| licensed IBIS model.
| 10.This license is subject to the laws of the state of Texas, USA, without
| regard for its conflicts of laws provisions.
[IBIS ver] 3.2
[File name] efr32xg23_qfn40_hfclkout.ibs
[File Rev] 1.0
[Date]  Oct 26, 2021
[Source] File originated at Silicon Labs Inc.
[Notes]  1. MIN TYP MAX information is based on Temperature and Voltage
   characteristics only.
   2. The model of I/O buffer has the mode of input, input w/ pull-
   down resistor, input w/ pull-up resistor, pushpull, wiredor,
   wiredor w/ pull-down resistor, wiredand, wiredand w/ pull-up
   resistor.
   3. Supply voltages modelled are 1.8V, 3.0V and 3.3V.
   4. Slew rate of buffer can be typ (sr4), min (sr0), max (sr7).
[Disclaimer]
| READ THE TERMS OF THIS LICENSE BEFORE USING THIS IBIS MODEL. IF YOU DO
| NOT ACCEPT THE TERMS OF THIS LICENSE, YOU ARE NOT PERMITTED TO USE THIS
| IBIS MODEL.
| Silicon Laboratories Inc. ("Silicon Labs") is the exclusive owner of this
| IBIS model,  and hereby grants to Licensee a limited, non-exclusive,
| worldwide, royalty-free, non-transferable, perpetual license to use this
| IBIS model, subject to the following terms and conditions:
| 1.If you are using this IBIS model for the benefit of your employer,
| then your acceptance of these terms will be considered an acceptance by
| your employer and your employer will be deemed to be the Licensee of this
| IBIS model.
| 2.Licensee is granted this license to use this IBIS model only for the
| purpose  modeling input/output buffers of Silicon Labs integrated circuits,
| and is not granted any rights to sell, load, rent, lease or license this
| IBIS model in whole or in part, or in modified form, to any third party.
| 3.Licensee may modify this IBIS model to suit its specific applications,
| but rights to derivative works and such modifications, including all
| intellectual property rights, shall belong exclusively to Silicon Labs. To
| the extent that Silicon Labs is not the owner of such modifications or
| derivatives, Licensee hereby grants to Silicon Labs a non-exclusive,
| worldwide, royalty-free, fully-transferable, assignable, perpetual license
| to use, copy, modify, make derivatives, sell, offer to sell, make, have
| made and sub-license such derivative and modifications in any manner, for
| any purpose, with no accounting to Licensee.
| 4.This IBIS model is provided on an "AS IS" basis and Silicon Labs makes
| no representations or warranties with respect to the information contained
| in this IBIS model.
| 5.SILICON LABS DISCLAIMS AND LICENSEE WAIVES ALL WARRANTIES, EXPRESS OR
| IMPLIED, INCLUDING WARRANTIES OF MERCHANTABILITY, NON-INFRINGEMENT AND
| FITNESS FOR A PARTICULAR PURPOSE.
| 6.The entire risk as to quality and performance is with Licensee.
| ACCORDINGLY, IN NO EVENT SHALL SILICON LABS BE LIABLE FOR ANY DAMAGES,
| WHETHER IN CONTRACT OR TORT, INCLUDING ANY LOST PROFITS OR OTHER INCIDENTAL,
| CONSEQUENTIAL, EXEMPLARY, OR PUNITIVE DAMAGES ARISING OUT OF THE USE OR
| APPLICATION OF THIS IBIS MODEL.
| 7.Silicon Labs reserves the right to make changes without notice to this
| IBIS model to improve reliability, function, or design.
| 8.Silicon Labs does not convey any license under patent rights or any other
| intellectual property rights, including those of third parties.
| 9.Silicon Labs is not obligated to provide maintenance or support for the
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[Copyright] Copyright 2021 Silicon Labs Inc.
|   Component 40nm General Purpose
[Component] Ocelot
[Manufacturer] Silicon Labs Inc.
[Package]
| QFN40
| variable   typ   min   max
R_pkg   0.467   0.424   0.495
L_pkg   1.57E-09	8.37E-10	2.02E-09
C_pkg   2.59E-13	1.87E-13	4.17E-13
[Pin]	signal_name	model_name	R_pin   L_pin   C_pin
1	PC00   gpio_lcd	0.477   1.72E-09	2.59E-13
2	PC01   gpio_lcd	0.466   1.55E-09	2.45E-13
3	PC02   gpio_lcd	0.456   1.38E-09	2.31E-13
4	PC03   gpio_lcd	0.454   1.34E-09	2.28E-13
5	PC04   gpio_lcd	0.452   1.31E-09	2.25E-13
6	PC05   gpio_lcd	0.458   1.42E-09	2.34E-13
7	PC06   gpio_lcd	0.470   1.61E-09	2.50E-13
8	HFCLKOUT	NC   0.453   1.32E-09	2.27E-13
9	HFXTAL_I	NC   0.455   1.36E-09	2.30E-13
10	HFXTAL_O	NC   0.463   1.49E-09	2.40E-13
11	RESETn   NC   0.463   1.49E-09	2.40E-13
12	RFVDD   NC   0.459   1.43E-09	2.35E-13
13	RFVSS   NC   0.424   8.37E-10	1.87E-13
14	SUBG_I1   NC   0.455   1.35E-09	2.29E-13
15	SUBG_I0   NC   0.456   1.37E-09	2.31E-13
16	SUBG_O1   NC   0.459   1.43E-09	2.35E-13
17	SUBG_O0   NC   0.464   1.51E-09	2.42E-13
18	PAVDD   NC   0.470   1.62E-09	2.50E-13
19	PB01   gpio_lcd	0.467   1.55E-09	2.45E-13
20	PB00   gpio_lcd	0.480   1.78E-09	2.63E-13
21	PA00   gpio_lcd	0.487   1.89E-09	2.72E-13
22	PA01   gpio_lcd	0.476   1.71E-09	2.58E-13
23	PA02   gpio_3v   0.472   1.64E-09	2.53E-13
24	PA03   gpio_3v   0.473   1.66E-09	2.54E-13
25	PA04   gpio_lcd	0.479   1.77E-09	2.62E-13
26	PA05   gpio_lcd	0.491   1.95E-09	2.78E-13
27	PA06   gpio_lcd	0.473   1.66E-09	2.54E-13
28	PA07   gpio_lcd	0.479   1.76E-09	2.62E-13
29	PA08   gpio_lcd	0.489   1.93E-09	2.76E-13
30	DECOUPLE	NC   0.495   2.02E-09	2.83E-13
31	VREGSW   NC   0.451   1.29E-09	4.17E-13
32	VREGVDD 	NC   0.446   1.21E-09	3.91E-13
33	VREGVSS   NC   0.442   1.15E-09	3.70E-13
34	DVDD   NC   0.477   1.73E-09	2.60E-13
35	AVDD   NC   0.475   1.70E-09	2.57E-13
36	IOVDD   NC   0.478   1.75E-09	2.61E-13
37	PD03   gpio_lcd	0.476   1.71E-09	2.58E-13
38	PD02   gpio_lcd	0.476   1.70E-09	2.58E-13
39	PD01   gpio_3v   0.477   1.73E-09	2.60E-13
40	PD00   gpio_3v   0.482   1.82E-09	2.67E-13
| End of package information
[Component]   gpio_lcd
[Manufacturer]   Silicon Labs Inc.
[Package]
|  variable   typ   min   max
R_pkg   0   0   0
L_pkg   0   0   0
C_pkg   0   0   0
[Pin]   signal_name   model_name   R_pin   L_pin   C_pin
vdd   vddio   POWER
pad   pad   gpio_lcd
gnd   gndio   GND
[Model Selector] gpio_lcd
lcd_input_1p8V_sr0  1.8V, input mode, MODEn=0/1, slew_rate=0, SLEWRATE[ALT]=0
lcd_input_1p8V_sr4  1.8V, input mode, MODEn=0/1, slew_rate=4, SLEWRATE[ALT]=4
lcd_input_1p8V_sr7  1.8V, input mode, MODEn=0/1, slew_rate=7, SLEWRATE[ALT]=7
lcd_input_3p0V_sr0  3.0V, input mode, MODEn=0/1, slew_rate=0, SLEWRATE[ALT]=0
lcd_input_3p0V_sr4  3.0V, input mode, MODEn=0/1, slew_rate=4, SLEWRATE[ALT]=4
lcd_input_3p0V_sr7  3.0V, input mode, MODEn=0/1, slew_rate=7, SLEWRATE[ALT]=7
lcd_input_3p3V_sr0  3.3V, input mode, MODEn=0/1, slew_rate=0, SLEWRATE[ALT]=0
lcd_input_3p3V_sr4  3.3V, input mode, MODEn=0/1, slew_rate=4, SLEWRATE[ALT]=4
lcd_input_3p3V_sr7  3.3V, input mode, MODEn=0/1, slew_rate=7, SLEWRATE[ALT]=7
lcd_inputpd_1p8V_sr0  1.8V, input mode with pull-down res, MODEn=2/3, slew_rate=0, SLEWRATE[ALT]=0
lcd_inputpd_1p8V_sr4  1.8V, input mode with pull-down res, MODEn=2/3, slew_rate=4, SLEWRATE[ALT]=4
lcd_inputpd_1p8V_sr7  1.8V, input mode with pull-down res, MODEn=2/3, slew_rate=7, SLEWRATE[ALT]=7
lcd_inputpd_3p0V_sr0  3.0V, input mode with pull-down res, MODEn=2/3, slew_rate=0, SLEWRATE[ALT]=0
lcd_inputpd_3p0V_sr4  3.0V, input mode with pull-down res, MODEn=2/3, slew_rate=4, SLEWRATE[ALT]=4
lcd_inputpd_3p0V_sr7  3.0V, input mode with pull-down res, MODEn=2/3, slew_rate=7, SLEWRATE[ALT]=7
lcd_inputpd_3p3V_sr0  3.3V, input mode with pull-down res, MODEn=2/3, slew_rate=0, SLEWRATE[ALT]=0
lcd_inputpd_3p3V_sr4  3.3V, input mode with pull-down res, MODEn=2/3, slew_rate=4, SLEWRATE[ALT]=4
lcd_inputpd_3p3V_sr7  3.3V, input mode with pull-down res, MODEn=2/3, slew_rate=7, SLEWRATE[ALT]=7
lcd_inputpu_1p8V_sr0  1.8V, input mode with pull-up res, MODEn=2/3, slew_rate=0, SLEWRATE[ALT]=0
lcd_inputpu_1p8V_sr4  1.8V, input mode with pull-up res, MODEn=2/3, slew_rate=4, SLEWRATE[ALT]=4
lcd_inputpu_1p8V_sr7  1.8V, input mode with pull-up res, MODEn=2/3, slew_rate=7, SLEWRATE[ALT]=7
lcd_inputpu_3p0V_sr0  3.0V, input mode with pull-up res, MODEn=2/3, slew_rate=0, SLEWRATE[ALT]=0
lcd_inputpu_3p0V_sr4  3.0V, input mode with pull-up res, MODEn=2/3, slew_rate=4, SLEWRATE[ALT]=4
lcd_inputpu_3p0V_sr7  3.0V, input mode with pull-up res, MODEn=2/3, slew_rate=7, SLEWRATE[ALT]=7
lcd_inputpu_3p3V_sr0  3.3V, input mode with pull-up res, MODEn=2/3, slew_rate=0, SLEWRATE[ALT]=0
lcd_inputpu_3p3V_sr4  3.3V, input mode with pull-up res, MODEn=2/3, slew_rate=4, SLEWRATE[ALT]=4
lcd_inputpu_3p3V_sr7  3.3V, input mode with pull-up res, MODEn=2/3, slew_rate=7, SLEWRATE[ALT]=7
lcd_pushpull_1p8V_sr0  1.8V, pushpull mode, MODEn=4/5, slew_rate=0, SLEWRATE[ALT]=0
lcd_pushpull_1p8V_sr4  1.8V, pushpull mode, MODEn=4/5, slew_rate=4, SLEWRATE[ALT]=4
lcd_pushpull_1p8V_sr7  1.8V, pushpull mode, MODEn=4/5, slew_rate=7, SLEWRATE[ALT]=7
lcd_pushpull_3p0V_sr0  3.0V, pushpull mode, MODEn=4/5, slew_rate=0, SLEWRATE[ALT]=0
lcd_pushpull_3p0V_sr4  3.0V, pushpull mode, MODEn=4/5, slew_rate=4, SLEWRATE[ALT]=4
lcd_pushpull_3p0V_sr7  3.0V, pushpull mode, MODEn=4/5, slew_rate=7, SLEWRATE[ALT]=7
lcd_pushpull_3p3V_sr0  3.3V, pushpull mode, MODEn=4/5, slew_rate=0, SLEWRATE[ALT]=0
lcd_pushpull_3p3V_sr4  3.3V, pushpull mode, MODEn=4/5, slew_rate=4, SLEWRATE[ALT]=4
lcd_pushpull_3p3V_sr7  3.3V, pushpull mode, MODEn=4/5, slew_rate=7, SLEWRATE[ALT]=7
lcd_wiredor_1p8V_sr0  1.8V, open-source mode, MODEn=6, slew_rate=0, SLEWRATE[ALT]=0
lcd_wiredor_1p8V_sr4  1.8V, open-source mode, MODEn=6, slew_rate=4, SLEWRATE[ALT]=4
lcd_wiredor_1p8V_sr7  1.8V, open-source mode, MODEn=6, slew_rate=7, SLEWRATE[ALT]=7
lcd_wiredor_3p0V_sr0  3.0V, open-source mode, MODEn=6, slew_rate=0, SLEWRATE[ALT]=0
lcd_wiredor_3p0V_sr4  3.0V, open-source mode, MODEn=6, slew_rate=4, SLEWRATE[ALT]=4
lcd_wiredor_3p0V_sr7  3.0V, open-source mode, MODEn=6, slew_rate=7, SLEWRATE[ALT]=7
lcd_wiredor_3p3V_sr0  3.3V, open-source mode, MODEn=6, slew_rate=0, SLEWRATE[ALT]=0
lcd_wiredor_3p3V_sr4  3.3V, open-source mode, MODEn=6, slew_rate=4, SLEWRATE[ALT]=4
lcd_wiredor_3p3V_sr7  3.3V, open-source mode, MODEn=6, slew_rate=7, SLEWRATE[ALT]=7
lcd_wiredorpd_1p8V_sr0  1.8V, open-source mode with pull-down res, MODEn=7, slew_rate=0, SLEWRATE[ALT]=0
lcd_wiredorpd_1p8V_sr4  1.8V, open-source mode with pull-down res, MODEn=7, slew_rate=4, SLEWRATE[ALT]=4
lcd_wiredorpd_1p8V_sr7  1.8V, open-source mode with pull-down res, MODEn=7, slew_rate=7, SLEWRATE[ALT]=7
lcd_wiredorpd_3p0V_sr0  3.0V, open-source mode with pull-down res, MODEn=7, slew_rate=0, SLEWRATE[ALT]=0
lcd_wiredorpd_3p0V_sr4  3.0V, open-source mode with pull-down res, MODEn=7, slew_rate=4, SLEWRATE[ALT]=4
lcd_wiredorpd_3p0V_sr7  3.0V, open-source mode with pull-down res, MODEn=7, slew_rate=7, SLEWRATE[ALT]=7
lcd_wiredorpd_3p3V_sr0  3.3V, open-source mode with pull-down res, MODEn=7, slew_rate=0, SLEWRATE[ALT]=0
lcd_wiredorpd_3p3V_sr4  3.3V, open-source mode with pull-down res, MODEn=7, slew_rate=4, SLEWRATE[ALT]=4
lcd_wiredorpd_3p3V_sr7  3.3V, open-source mode with pull-down res, MODEn=7, slew_rate=7, SLEWRATE[ALT]=7
lcd_wiredand_1p8V_sr0  1.8V, open-drain mode, MODEn=8/9/12/13, slew_rate=0, SLEWRATE[ALT]=0
lcd_wiredand_1p8V_sr4  1.8V, open-drain mode, MODEn=8/9/12/13, slew_rate=4, SLEWRATE[ALT]=4
lcd_wiredand_1p8V_sr7  1.8V, open-drain mode, MODEn=8/9/12/13, slew_rate=7, SLEWRATE[ALT]=7
lcd_wiredand_3p0V_sr0  3.0V, open-drain mode, MODEn=8/9/12/13, slew_rate=0, SLEWRATE[ALT]=0
lcd_wiredand_3p0V_sr4  3.0V, open-drain mode, MODEn=8/9/12/13, slew_rate=4, SLEWRATE[ALT]=4
lcd_wiredand_3p0V_sr7  3.0V, open-drain mode, MODEn=8/9/12/13, slew_rate=7, SLEWRATE[ALT]=7
lcd_wiredand_3p3V_sr0  3.3V, open-drain mode, MODEn=8/9/12/13, slew_rate=0, SLEWRATE[ALT]=0
lcd_wiredand_3p3V_sr4  3.3V, open-drain mode, MODEn=8/9/12/13, slew_rate=4, SLEWRATE[ALT]=4
lcd_wiredand_3p3V_sr7  3.3V, open-drain mode, MODEn=8/9/12/13, slew_rate=7, SLEWRATE[ALT]=7
lcd_wiredandpu_1p8V_sr0  1.8V, open-drain mode with pull-up res, MODEn=10/11/14/15, slew_rate=0, SLEWRATE[ALT]=0
lcd_wiredandpu_1p8V_sr4  1.8V, open-drain mode with pull-up res, MODEn=10/11/14/15, slew_rate=4, SLEWRATE[ALT]=4
lcd_wiredandpu_1p8V_sr7  1.8V, open-drain mode with pull-up res, MODEn=10/11/14/15, slew_rate=7, SLEWRATE[ALT]=7
lcd_wiredandpu_3p0V_sr0  3.0V, open-drain mode with pull-up res, MODEn=10/11/14/15, slew_rate=0, SLEWRATE[ALT]=0
lcd_wiredandpu_3p0V_sr4  3.0V, open-drain mode with pull-up res, MODEn=10/11/14/15, slew_rate=4, SLEWRATE[ALT]=4
lcd_wiredandpu_3p0V_sr7  3.0V, open-drain mode with pull-up res, MODEn=10/11/14/15, slew_rate=7, SLEWRATE[ALT]=7
lcd_wiredandpu_3p3V_sr0  3.3V, open-drain mode with pull-up res, MODEn=10/11/14/15, slew_rate=0, SLEWRATE[ALT]=0
lcd_wiredandpu_3p3V_sr4  3.3V, open-drain mode with pull-up res, MODEn=10/11/14/15, slew_rate=4, SLEWRATE[ALT]=4
lcd_wiredandpu_3p3V_sr7  3.3V, open-drain mode with pull-up res, MODEn=10/11/14/15, slew_rate=7, SLEWRATE[ALT]=7
[Component]   gpio_3v
[Manufacturer]   Silicon Labs Inc.
[Package]
|  variable   typ   min   max
R_pkg   0   0   0
L_pkg   0   0   0
C_pkg   0   0   0
[Pin]   signal_name   model_name   R_pin   L_pin   C_pin
vdd   vddio   POWER
pad   pad   gpio_3v
gnd   gndio   GND
[Model Selector] gpio_3v
3v_input_1p8V_sr0  1.8V, input mode, MODEn=0/1, slew_rate=0, SLEWRATE[ALT]=0
3v_input_1p8V_sr4  1.8V, input mode, MODEn=0/1, slew_rate=4, SLEWRATE[ALT]=4
3v_input_1p8V_sr7  1.8V, input mode, MODEn=0/1, slew_rate=7, SLEWRATE[ALT]=7
3v_input_3p0V_sr0  3.0V, input mode, MODEn=0/1, slew_rate=0, SLEWRATE[ALT]=0
3v_input_3p0V_sr4  3.0V, input mode, MODEn=0/1, slew_rate=4, SLEWRATE[ALT]=4
3v_input_3p0V_sr7  3.0V, input mode, MODEn=0/1, slew_rate=7, SLEWRATE[ALT]=7
3v_input_3p3V_sr0  3.3V, input mode, MODEn=0/1, slew_rate=0, SLEWRATE[ALT]=0
3v_input_3p3V_sr4  3.3V, input mode, MODEn=0/1, slew_rate=4, SLEWRATE[ALT]=4
3v_input_3p3V_sr7  3.3V, input mode, MODEn=0/1, slew_rate=7, SLEWRATE[ALT]=7
3v_inputpd_1p8V_sr0  1.8V, input mode with pull-down res, MODEn=2/3, slew_rate=0, SLEWRATE[ALT]=0
3v_inputpd_1p8V_sr4  1.8V, input mode with pull-down res, MODEn=2/3, slew_rate=4, SLEWRATE[ALT]=4
3v_inputpd_1p8V_sr7  1.8V, input mode with pull-down res, MODEn=2/3, slew_rate=7, SLEWRATE[ALT]=7
3v_inputpd_3p0V_sr0  3.0V, input mode with pull-down res, MODEn=2/3, slew_rate=0, SLEWRATE[ALT]=0
3v_inputpd_3p0V_sr4  3.0V, input mode with pull-down res, MODEn=2/3, slew_rate=4, SLEWRATE[ALT]=4
3v_inputpd_3p0V_sr7  3.0V, input mode with pull-down res, MODEn=2/3, slew_rate=7, SLEWRATE[ALT]=7
3v_inputpd_3p3V_sr0  3.3V, input mode with pull-down res, MODEn=2/3, slew_rate=0, SLEWRATE[ALT]=0
3v_inputpd_3p3V_sr4  3.3V, input mode with pull-down res, MODEn=2/3, slew_rate=4, SLEWRATE[ALT]=4
3v_inputpd_3p3V_sr7  3.3V, input mode with pull-down res, MODEn=2/3, slew_rate=7, SLEWRATE[ALT]=7
3v_inputpu_1p8V_sr0  1.8V, input mode with pull-up res, MODEn=2/3, slew_rate=0, SLEWRATE[ALT]=0
3v_inputpu_1p8V_sr4  1.8V, input mode with pull-up res, MODEn=2/3, slew_rate=4, SLEWRATE[ALT]=4
3v_inputpu_1p8V_sr7  1.8V, input mode with pull-up res, MODEn=2/3, slew_rate=7, SLEWRATE[ALT]=7
3v_inputpu_3p0V_sr0  3.0V, input mode with pull-up res, MODEn=2/3, slew_rate=0, SLEWRATE[ALT]=0
3v_inputpu_3p0V_sr4  3.0V, input mode with pull-up res, MODEn=2/3, slew_rate=4, SLEWRATE[ALT]=4
3v_inputpu_3p0V_sr7  3.0V, input mode with pull-up res, MODEn=2/3, slew_rate=7, SLEWRATE[ALT]=7
3v_inputpu_3p3V_sr0  3.3V, input mode with pull-up res, MODEn=2/3, slew_rate=0, SLEWRATE[ALT]=0
3v_inputpu_3p3V_sr4  3.3V, input mode with pull-up res, MODEn=2/3, slew_rate=4, SLEWRATE[ALT]=4
3v_inputpu_3p3V_sr7  3.3V, input mode with pull-up res, MODEn=2/3, slew_rate=7, SLEWRATE[ALT]=7
3v_pushpull_1p8V_sr0  1.8V, pushpull mode, MODEn=4/5, slew_rate=0, SLEWRATE[ALT]=0
3v_pushpull_1p8V_sr4  1.8V, pushpull mode, MODEn=4/5, slew_rate=4, SLEWRATE[ALT]=4
3v_pushpull_1p8V_sr7  1.8V, pushpull mode, MODEn=4/5, slew_rate=7, SLEWRATE[ALT]=7
3v_pushpull_3p0V_sr0  3.0V, pushpull mode, MODEn=4/5, slew_rate=0, SLEWRATE[ALT]=0
3v_pushpull_3p0V_sr4  3.0V, pushpull mode, MODEn=4/5, slew_rate=4, SLEWRATE[ALT]=4
3v_pushpull_3p0V_sr7  3.0V, pushpull mode, MODEn=4/5, slew_rate=7, SLEWRATE[ALT]=7
3v_pushpull_3p3V_sr0  3.3V, pushpull mode, MODEn=4/5, slew_rate=0, SLEWRATE[ALT]=0
3v_pushpull_3p3V_sr4  3.3V, pushpull mode, MODEn=4/5, slew_rate=4, SLEWRATE[ALT]=4
3v_pushpull_3p3V_sr7  3.3V, pushpull mode, MODEn=4/5, slew_rate=7, SLEWRATE[ALT]=7
3v_wiredor_1p8V_sr0  1.8V, open-source mode, MODEn=6, slew_rate=0, SLEWRATE[ALT]=0
3v_wiredor_1p8V_sr4  1.8V, open-source mode, MODEn=6, slew_rate=4, SLEWRATE[ALT]=4
3v_wiredor_1p8V_sr7  1.8V, open-source mode, MODEn=6, slew_rate=7, SLEWRATE[ALT]=7
3v_wiredor_3p0V_sr0  3.0V, open-source mode, MODEn=6, slew_rate=0, SLEWRATE[ALT]=0
3v_wiredor_3p0V_sr4  3.0V, open-source mode, MODEn=6, slew_rate=4, SLEWRATE[ALT]=4
3v_wiredor_3p0V_sr7  3.0V, open-source mode, MODEn=6, slew_rate=7, SLEWRATE[ALT]=7
3v_wiredor_3p3V_sr0  3.3V, open-source mode, MODEn=6, slew_rate=0, SLEWRATE[ALT]=0
3v_wiredor_3p3V_sr4  3.3V, open-source mode, MODEn=6, slew_rate=4, SLEWRATE[ALT]=4
3v_wiredor_3p3V_sr7  3.3V, open-source mode, MODEn=6, slew_rate=7, SLEWRATE[ALT]=7
3v_wiredorpd_1p8V_sr0  1.8V, open-source mode with pull-down res, MODEn=7, slew_rate=0, SLEWRATE[ALT]=0
3v_wiredorpd_1p8V_sr4  1.8V, open-source mode with pull-down res, MODEn=7, slew_rate=4, SLEWRATE[ALT]=4
3v_wiredorpd_1p8V_sr7  1.8V, open-source mode with pull-down res, MODEn=7, slew_rate=7, SLEWRATE[ALT]=7
3v_wiredorpd_3p0V_sr0  3.0V, open-source mode with pull-down res, MODEn=7, slew_rate=0, SLEWRATE[ALT]=0
3v_wiredorpd_3p0V_sr4  3.0V, open-source mode with pull-down res, MODEn=7, slew_rate=4, SLEWRATE[ALT]=4
3v_wiredorpd_3p0V_sr7  3.0V, open-source mode with pull-down res, MODEn=7, slew_rate=7, SLEWRATE[ALT]=7
3v_wiredorpd_3p3V_sr0  3.3V, open-source mode with pull-down res, MODEn=7, slew_rate=0, SLEWRATE[ALT]=0
3v_wiredorpd_3p3V_sr4  3.3V, open-source mode with pull-down res, MODEn=7, slew_rate=4, SLEWRATE[ALT]=4
3v_wiredorpd_3p3V_sr7  3.3V, open-source mode with pull-down res, MODEn=7, slew_rate=7, SLEWRATE[ALT]=7
3v_wiredand_1p8V_sr0  1.8V, open-drain mode, MODEn=8/9/12/13, slew_rate=0, SLEWRATE[ALT]=0
3v_wiredand_1p8V_sr4  1.8V, open-drain mode, MODEn=8/9/12/13, slew_rate=4, SLEWRATE[ALT]=4
3v_wiredand_1p8V_sr7  1.8V, open-drain mode, MODEn=8/9/12/13, slew_rate=7, SLEWRATE[ALT]=7
3v_wiredand_3p0V_sr0  3.0V, open-drain mode, MODEn=8/9/12/13, slew_rate=0, SLEWRATE[ALT]=0
3v_wiredand_3p0V_sr4  3.0V, open-drain mode, MODEn=8/9/12/13, slew_rate=4, SLEWRATE[ALT]=4
3v_wiredand_3p0V_sr7  3.0V, open-drain mode, MODEn=8/9/12/13, slew_rate=7, SLEWRATE[ALT]=7
3v_wiredand_3p3V_sr0  3.3V, open-drain mode, MODEn=8/9/12/13, slew_rate=0, SLEWRATE[ALT]=0
3v_wiredand_3p3V_sr4  3.3V, open-drain mode, MODEn=8/9/12/13, slew_rate=4, SLEWRATE[ALT]=4
3v_wiredand_3p3V_sr7  3.3V, open-drain mode, MODEn=8/9/12/13, slew_rate=7, SLEWRATE[ALT]=7
3v_wiredandpu_1p8V_sr0  1.8V, open-drain mode with pull-up res, MODEn=10/11/14/15, slew_rate=0, SLEWRATE[ALT]=0
3v_wiredandpu_1p8V_sr4  1.8V, open-drain mode with pull-up res, MODEn=10/11/14/15, slew_rate=4, SLEWRATE[ALT]=4
3v_wiredandpu_1p8V_sr7  1.8V, open-drain mode with pull-up res, MODEn=10/11/14/15, slew_rate=7, SLEWRATE[ALT]=7
3v_wiredandpu_3p0V_sr0  3.0V, open-drain mode with pull-up res, MODEn=10/11/14/15, slew_rate=0, SLEWRATE[ALT]=0
3v_wiredandpu_3p0V_sr4  3.0V, open-drain mode with pull-up res, MODEn=10/11/14/15, slew_rate=4, SLEWRATE[ALT]=4
3v_wiredandpu_3p0V_sr7  3.0V, open-drain mode with pull-up res, MODEn=10/11/14/15, slew_rate=7, SLEWRATE[ALT]=7
3v_wiredandpu_3p3V_sr0  3.3V, open-drain mode with pull-up res, MODEn=10/11/14/15, slew_rate=0, SLEWRATE[ALT]=0
3v_wiredandpu_3p3V_sr4  3.3V, open-drain mode with pull-up res, MODEn=10/11/14/15, slew_rate=4, SLEWRATE[ALT]=4
3v_wiredandpu_3p3V_sr7  3.3V, open-drain mode with pull-up res, MODEn=10/11/14/15, slew_rate=7, SLEWRATE[ALT]=7
| Models and submodels in the file (144): lcd_input_1p8_sr0 (Input), lcd_input_1p8_sr4 (Input), lcd_input_1p8_sr7 (Input), lcd_input_3p0_sr0 (Input), lcd_input_3p0_sr4 (Input), lcd_input_3p0_sr7 (Input), lcd_input_3p3_sr0 (Input), lcd_input_3p3_sr4 (Input), lcd_input_3p3_sr7 (Input), lcd_inputpd_1p8_sr0 (Input), lcd_inputpd_1p8_sr4 (Input), lcd_inputpd_1p8_sr7 (Input), lcd_inputpd_3p0_sr0 (Input), lcd_inputpd_3p0_sr4 (Input), lcd_inputpd_3p0_sr7 (Input), lcd_inputpd_3p3_sr0 (Input), lcd_inputpd_3p3_sr4 (Input), lcd_inputpd_3p3_sr7 (Input), lcd_inputpu_1p8_sr0 (Input), lcd_inputpu_1p8_sr4 (Input), lcd_inputpu_1p8_sr7 (Input), lcd_inputpu_3p0_sr0 (Input), lcd_inputpu_3p0_sr4 (Input), lcd_inputpu_3p0_sr7 (Input), lcd_inputpu_3p3_sr0 (Input), lcd_inputpu_3p3_sr4 (Input), lcd_inputpu_3p3_sr7 (Input), lcd_pushpull_1p8_sr0 (3-state), lcd_pushpull_1p8_sr4 (3-state), lcd_pushpull_1p8_sr7 (3-state), lcd_pushpull_3p0_sr0 (3-state), lcd_pushpull_3p0_sr4 (3-state), lcd_pushpull_3p0_sr7 (3-state), lcd_pushpull_3p3_sr0 (3-state), lcd_pushpull_3p3_sr4 (3-state), lcd_pushpull_3p3_sr7 (3-state), lcd_wiredor_1p8_sr0 (Output), lcd_wiredor_1p8_sr4 (Output), lcd_wiredor_1p8_sr7 (Output), lcd_wiredor_3p0_sr0 (Output), lcd_wiredor_3p0_sr4 (Output), lcd_wiredor_3p0_sr7 (Output), lcd_wiredor_3p3_sr0 (Output), lcd_wiredor_3p3_sr4 (Output), lcd_wiredor_3p3_sr7 (Output), lcd_wiredorpd_1p8_sr0 (Output), lcd_wiredorpd_1p8_sr4 (Output), lcd_wiredorpd_1p8_sr7 (Output), lcd_wiredorpd_3p0_sr0 (Output), lcd_wiredorpd_3p0_sr4 (Output), lcd_wiredorpd_3p0_sr7 (Output), lcd_wiredorpd_3p3_sr0 (Output), lcd_wiredorpd_3p3_sr4 (Output), lcd_wiredorpd_3p3_sr7 (Output), lcd_wiredand_1p8_sr0 (Output), lcd_wiredand_1p8_sr4 (Output), lcd_wiredand_1p8_sr7 (Output), lcd_wiredand_3p0_sr0 (Output), lcd_wiredand_3p0_sr4 (Output), lcd_wiredand_3p0_sr7 (Output), lcd_wiredand_3p3_sr0 (Output), lcd_wiredand_3p3_sr4 (Output), lcd_wiredand_3p3_sr7 (Output), lcd_wiredandpu_1p8_sr0 (Output), lcd_wiredandpu_1p8_sr4 (Output), lcd_wiredandpu_1p8_sr7 (Output), lcd_wiredandpu_3p0_sr0 (Output), lcd_wiredandpu_3p0_sr4 (Output), lcd_wiredandpu_3p0_sr7 (Output), lcd_wiredandpu_3p3_sr0 (Output), lcd_wiredandpu_3p3_sr4 (Output), lcd_wiredandpu_3p3_sr7 (Output), 3v_input_1p8_sr0 (Input), 3v_input_1p8_sr4 (Input), 3v_input_1p8_sr7 (Input), 3v_input_3p0_sr0 (Input), 3v_input_3p0_sr4 (Input), 3v_input_3p0_sr7 (Input), 3v_input_3p3_sr0 (Input), 3v_input_3p3_sr4 (Input)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
